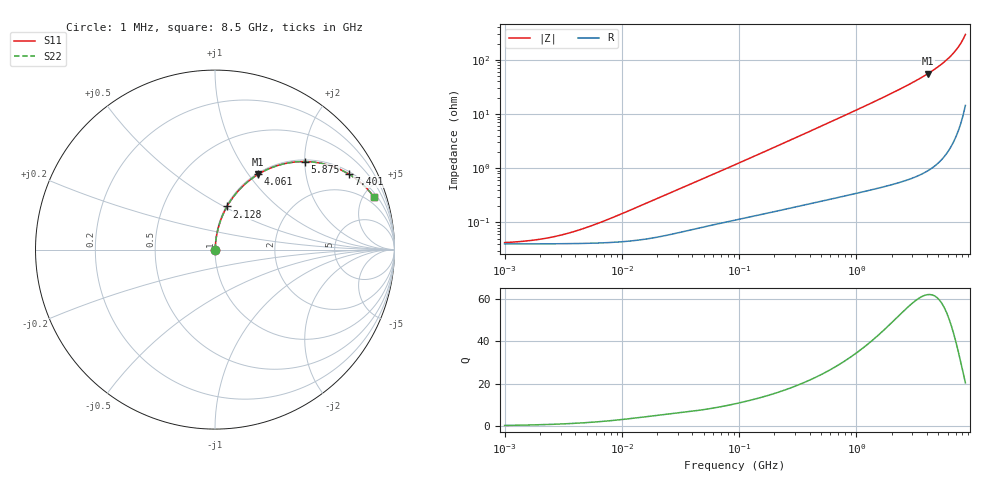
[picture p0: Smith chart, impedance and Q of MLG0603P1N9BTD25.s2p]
! S-Parameter Data Generated by TDK Corporation
! Copyright(C) 2025 TDK Corporation.
! All Rights Reserved.
! TDK P/N: MLG0603P1N9BTD25 (SMD / SMT Inductor (Coil))
! Property: L=1.9nH at 500MHz
! Size(LxWxT): 0.6x0.3x0.3mm
! Model Type: s2p (Touchstone File Format Version 1.0)
! Frequency: DC=Yes Start=1MHz Stop=8500MHz 198points Log-sweep
! Model Generated on Feb. 6, 2025
! Terms and conditions regarding TDK Simulation Models:
! 1)This simulation model is being provided solely for informational
!  purposes. Please refer to the specifications of the products in
!  terms of detailed characteristics of such products.
! 2)In no event shall TDK Corporation of any of its subsidiaries be
!  liable for any loss or damage arising, directly or indirectly,
!  from any information contained in this simulation model, including,
!  but not limited to loss or damages arising from any inaccuracies,
!  omissions or errors in connection with such information.
! 3)Any and all copyrights on this simulation model are owned by
!  TDK Corporation.  Duplication or redistribution of this simulation
!  model without prior written permission from TDK Corporation
!  is prohibited.
! 4)This simulation model is subject to any modification or change
!  without any prior notice.
! 5)Neither TDK Corporation nor any of its subsidiaries shall make any
!  warranty, express or implied, including but not limited to the
!  correctness, implied warranties of merchantability and fitness for
!  a particular purpose with respect to this simulation models.
! 6)The use of this simulation model shall be deemed to have consented
!  to the terms and conditions hereof.
! Port Assignments:
!  1 ---@@@--- 2
! Applicable Conditions:
!  Temperature = 25 degC
!  DC Bias Current = 0 A
!  Small Signal Operation
# Hz S MA R 50
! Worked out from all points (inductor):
!   197 points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, 1 MHz to 8.5 GHz, reference 50 ohm
!   read as one part in series: L = 2.19 nH near 9.602 MHz
!   highest Q = 62.1 at 4.061 GHz (marker M1), where L = 2.18 nH
!   S11 on the Smith chart (normalised r, x): 1 MHz: 1.00, +0.00; 2.128 GHz: 1.01, +0.52; 4.061 GHz: 1.02, +1.11; 5.875 GHz: 1.04, +2.00; 7.401 GHz: 1.10, +3.47; 8.5 GHz: 1.29, +5.90
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1000000  0.0004237 19.1  0.9996 -0.0  0.9996 -0.0  0.0004237 19.1
1515069  0.0004527 27.7  0.9996 -0.0  0.9996 -0.0  0.0004527 27.7
2191881  0.0005041 37.1  0.9996 -0.0  0.9996 -0.0  0.0005041 37.1
3171038  0.0005974 47.4  0.9996 -0.0  0.9996 -0.0  0.0005974 47.4
4587603  0.0007561 57.3  0.9996 -0.0  0.9996 -0.0  0.0007561 57.3
8360083  0.001232 69.6  0.9996 -0.1  0.9996 -0.1  0.001232 69.6
2.10461e7  0.0029 79.0  0.9995 -0.2  0.9995 -0.2  0.0029 79.0
9.219544e7  0.0116 83.9  0.9988 -0.7  0.9988 -0.7  0.0116 83.9
4.229561e8  0.05051 84.5  0.9965 -2.9  0.9965 -2.9  0.05051 84.5
9.708683e8  0.1143 81.8  0.9901 -6.6  0.9901 -6.6  0.1143 81.8
1.404574e9  0.1648 79.1  0.9823 -9.5  0.9823 -9.5  0.1648 79.1
1.940355e9  0.2276 75.7  0.969 -13.2  0.969 -13.2  0.2276 75.7
2.128028e9  0.2498 74.4  0.9633 -14.5  0.9633 -14.5  0.2498 74.4
3.07866e9  0.3635 67.7  0.9254 -21.3  0.9254 -21.3  0.3635 67.7
3.535948e9  0.4189 64.3  0.9012 -24.8  0.9012 -24.8  0.4189 64.3
4.061159e9  0.4831 60.2  0.8678 -28.9  0.8678 -28.9  0.4831 60.2
4.884749e9  0.5836 53.4  0.8025 -35.7  0.8025 -35.7  0.5836 53.4
5.87536e9  0.7006 44.5  0.7006 -44.5  0.7006 -44.5  0.7006 44.5
6.748056e9  0.7948 36.1  0.589 -52.6  0.589 -52.6  0.7948 36.1
7.400733e9  0.8558 29.6  0.4935 -58.8  0.4935 -58.8  0.8558 29.6
8.116539e9  0.9104 22.3  0.3796 -65.5  0.3796 -65.5  0.9104 22.3
8.5e9  0.9334 18.4  0.3161 -68.8  0.3161 -68.8  0.9334 18.4
